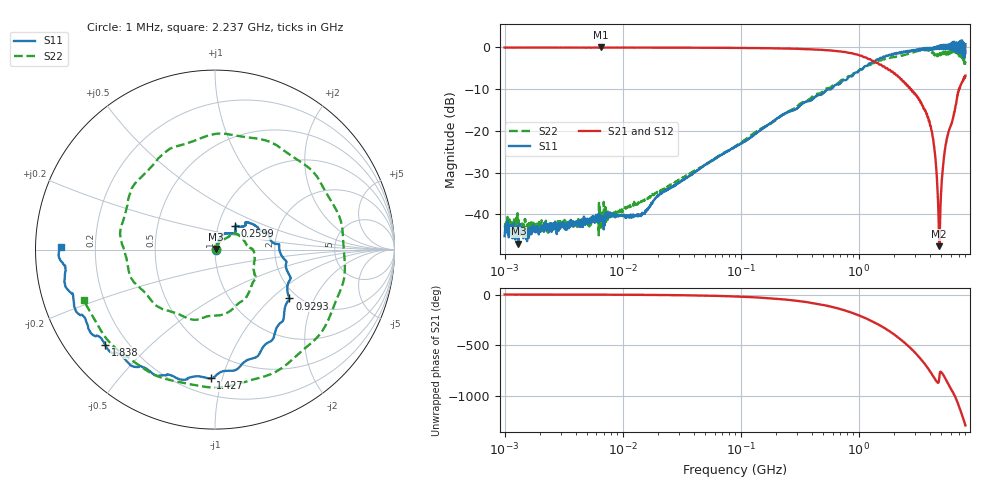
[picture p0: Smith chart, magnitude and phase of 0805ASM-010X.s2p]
!s-Parameter Generated by FASTRON Sdn. Bhd.
!FASTRON P/N : 0805ASM-010X
!Keysight Technologies: E5071C_MY46733604_B.14.02
!Date: Fri Jun 19 14:47:25 2026
!Version  :Rev00  Fri Jun 19 14:47:25 2026
!Data & Calibration Information:
!Freq  S11:SOLT2(ON)  S21:SOLT2(ON)  S12:SOLT2(ON)  S22:SOLT2(ON)
!PortZ  Port1:50+j0  Port2:50+j0
!When reading reference impedance value at option line is always used.
! Remarks : This data is being provided solely for informational purposes.
# Hz S dB R 50
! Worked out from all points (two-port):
!   1601 points, 1 MHz to 8 GHz, reference 50 ohm
!   highest |S21| = -0.04 dB at 6.532 MHz (marker M1); lowest = -47.6 dB at 4.801 GHz (marker M2)
!   |S21| within 3 dB of the highest: start of sweep to 1.272 GHz
!   lowest |S11| = -47.0 dB at 1.31 MHz (marker M3), VSWR 1.01, Z = 50.3 + j0.325 ohm
!   |S11| at or under -10 dB: start of sweep to 581.7 MHz
!   |S22| runs from -45.0 to -0.4 dB; largest |S21 - S12| = 0.016
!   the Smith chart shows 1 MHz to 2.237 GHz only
!   S11 on the Smith chart (normalised r, x): 1 MHz: 1.01, +0.00; 259.9 MHz: 1.20, +0.32; 929.3 MHz: 1.81, -1.31; 1.427 GHz: 0.31, -0.92; 1.838 GHz: 0.12, -0.37; 2.237 GHz: 0.08, +0.01
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1000000  -45.20 4.6  -0.07 -0.3  -0.06 -0.3  -42.80 6.4
1310238  -47.00 46.3  -0.08 -0.2  -0.10 -0.3  -41.30 -9.3
4479405  -42.10 23.0  -0.08 -1.0  -0.06 -1.1  -42.40 26.1
6531720  -41.10 39.2  -0.04 -1.4  -0.08 -1.5  -43.20 50.8
2.00676e7  -35.40 56.2  -0.08 -4.4  -0.09 -4.3  -34.60 56.7
8.994653e7  -23.80 66.3  -0.14 -19.1  -0.14 -19.0  -23.70 52.5
2.598545e8  -15.30 49.5  -0.32 -54.0  -0.32 -54.0  -15.20 12.9
4.006501e8  -12.50 40.0  -0.49 -82.8  -0.49 -82.8  -11.90 -30.5
9.292726e8  -6.09 -33.3  -1.64 169.0  -1.63 169.0  -6.10 -166.0
1.426888e9  -2.88 -92.0  -3.70 71.9  -3.71 71.7  -3.45 55.9
1.7949e9  -1.86 -134.0  -5.44 3.5  -5.43 3.1  -2.49 -40.1
1.83751e9  -1.84 -139.0  -5.42 -5.2  -5.45 -5.5  -2.56 -50.9
2.237469e9  -1.33 179.0  -7.40 -79.5  -7.43 -79.6  -2.11 -159.0
2.736325e9  -1.01 121.0  -10.00 -168.0  -10.00 -168.0  -1.43 79.2
3.446699e9  -0.51 52.9  -13.90 67.3  -13.90 67.2  -0.73 -104.0
4.115571e9  -0.63 -27.8  -19.80 -55.6  -19.70 -56.2  -1.07 93.8
4.800505e9  -0.43 -92.3  -47.60 -109.0  -47.40 -109.0  -2.03 -95.7
5.528293e9  0.53 -161.0  -22.30 -126.0  -22.40 -126.0  -1.27 91.6
6.226476e9  1.28 151.0  -17.40 124.0  -17.50 123.0  -0.42 -81.0
6.72769e9  1.12 101.0  -12.70 44.4  -12.90 43.8  -0.59 177.0
7.383122e9  0.52 24.0  -8.73 -84.4  -8.71 -84.7  -1.83 -15.8
8e9  0.75 -36.0  -6.77 150.0  -6.72 150.0  -3.36 179.0
